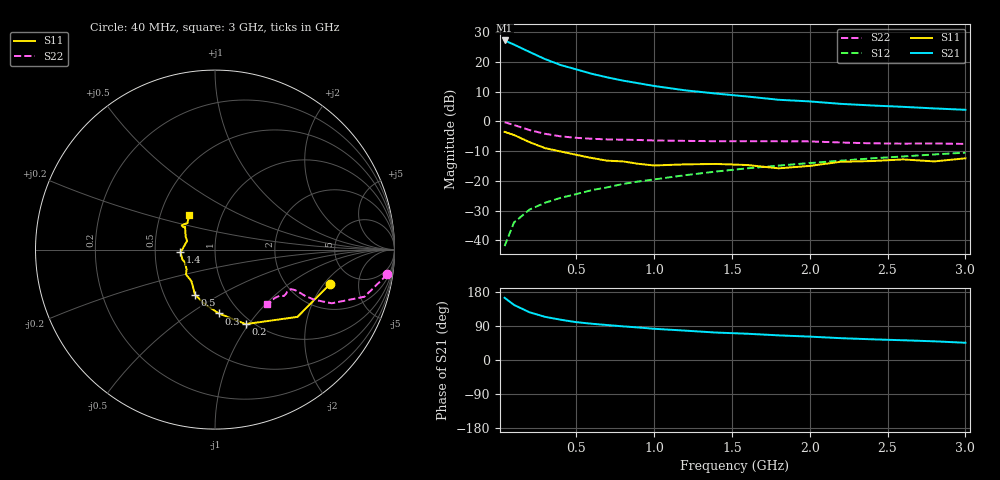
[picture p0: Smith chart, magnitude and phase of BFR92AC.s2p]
! Filename:  BFR92AC.S2P  Version:  2.0
! Philips part #: BFR92A  Date: May 1990
! Bias condition: Vce=5V, Ic=10mA
#  MHz  S  MA  R  50
! Freq  S11  S21  S12  S22  !GUM [dB]
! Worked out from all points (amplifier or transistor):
!   21 points, 40 MHz to 3 GHz, reference 50 ohm
!   highest |S21| = 27.2 dB at 40 MHz (marker M1)
!   |S21| within 3 dB of that: start of sweep to 165.1 MHz
!   unconditionally stable (mu >= 1): 947.1 MHz to 2.494 GHz
!   at 300 MHz: K = 0.71, MSG = 24.2 dB, |S12| = -27.3 dB
!   at 1 GHz: K = 1.02, MAG = 14.9 dB, |S12| = -19.5 dB
!   at 3 GHz: K = 0.98, MSG = 7.2 dB, |S12| = -10.5 dB
!   S11 on the Smith chart (normalised r, x): 40 MHz: 3.34, -2.31; 200 MHz: 0.93, -0.97; 300 MHz: 0.80, -0.65; 500 MHz: 0.71, -0.39; 1.4 GHz: 0.68, -0.02; 3 GHz: 0.70, +0.28
40  0.669 -16.6  23.02 164.2  0.008 79.9  0.97 -8.2
100  0.593 -39.2  19.63 145.4  0.02 72.1  0.873 -17.5
200  0.449 -67.6  14.75 125.9  0.033 68.7  0.716 -24.7
300  0.356 -86.7  11.18 113.9  0.043 66.2  0.62 -26.8
400  0.313 -99.2  8.899 106.3  0.052 68.0  0.562 -27.2
500  0.275 -113.9  7.512 99.9  0.06 67.4  0.531 -26.9
600  0.243 -120.1  6.336 95.7  0.07 69.7  0.512 -26.9
700  0.219 -127.0  5.513 92.2  0.078 71.3  0.499 -26.9
800  0.213 -139.5  4.868 88.8  0.089 72.4  0.494 -27.0
900  0.194 -144.7  4.391 85.8  0.098 72.5  0.488 -27.2
1000  0.182 -156.2  3.953 82.4  0.106 73.1  0.479 -27.4
1200  0.19 -163.4  3.339 77.5  0.125 73.5  0.472 -28.3
1400  0.193 -175.5  2.945 72.4  0.144 73.3  0.465 -30.1
1600  0.185 -179.0  2.626 69.3  0.163 73.6  0.466 -31.4
1800  0.163 163.1  2.316 65.0  0.181 73.3  0.465 -32.8
2000  0.179 156.0  2.174 61.7  0.2 72.6  0.462 -34.0
2200  0.21 142.6  1.977 57.6  0.219 72.5  0.443 -35.4
2400  0.216 144.8  1.857 54.6  0.24 71.1  0.429 -38.9
2600  0.23 143.8  1.762 52.1  0.258 70.5  0.424 -42.4
2800  0.213 136.1  1.657 49.3  0.279 70.0  0.427 -44.9
3000  0.24 127.1  1.571 45.5  0.299 68.6  0.419 -46.0
